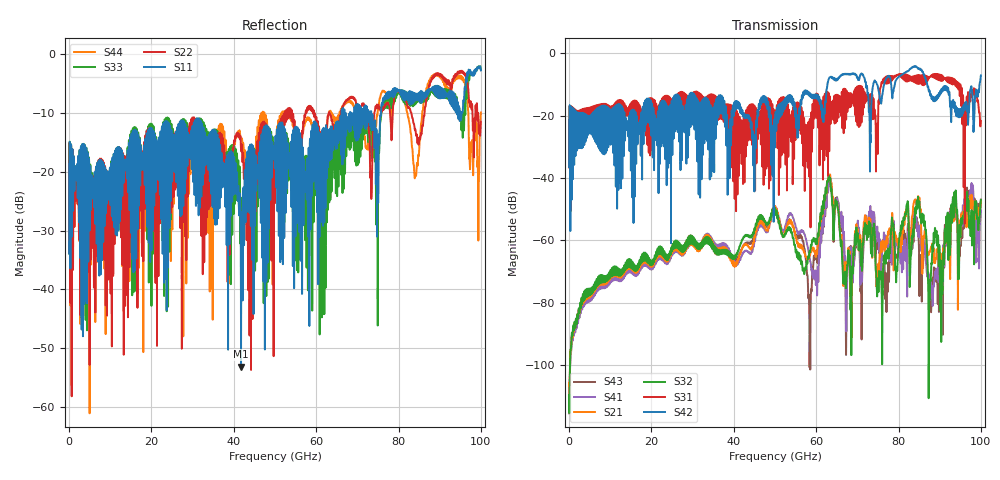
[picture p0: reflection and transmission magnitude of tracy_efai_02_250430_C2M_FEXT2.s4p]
!! PART DESCRIPTION: TE 224G+ VSR Channel- Chip to module, IO connector to CPC(Co-packaged connector) through over the board cable
!! CHANNEL DESCRIPTION: Module trace -> Mated IO 224G+ Connector -> Internal Cable Termination -> 30AWG 300mm Cable -> Cable
!!  termination + CPC connector(No footprint or package included)
!! MODEL REVISION:  Rev 3, Created on April 25, 2025
!! MODEL STATUS: Development
!! MODEL GEOMETRY: 8 Pair Channel
!! MODEL FREQUENCY RANGE: 0 GHz to 100 GHz in 10.00 MHz frequency steps
!! MODEL EDGE RATE LIMITATION: 5ps (Using conservative 0.5/Fmax rule of thumb)
!! PORT DEFINITIONS:
!! Port  1  ----->  Module Side  -->  Host Side, A Row  <-----  Port  2
!! Port  3  ----->  Module Side  -->  Host Side, A Row  <-----  Port  4
# GHz S MA R 45
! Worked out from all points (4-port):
!   10000 points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, 10 MHz to 100 GHz, reference 45 ohm
!   strongest paths, dB at 10 MHz, 25.01 GHz, 50.01 GHz, 75.01 GHz, 100 GHz:
!     S42: -36.5, -18.1, -28.3, -11.1, -7.2
!     S31: -36.7, -17.7, -20.3, -22.6, -21.7
!     S32: -115.0, -63.6, -49.7, -72.5, -47.1
!     S21: -112.4, -64.2, -49.2, -71.6, -47.8
!     S41: -115.1, -64.9, -49.3, -60.3, -50.4
!     S43: -115.4, -64.4, -49.9, -62.8, -46.9
!   lowest |S11| = -53.2 dB at 41.76 GHz (marker M1), VSWR 1.00, Z = 44.9 + j0.179 ohm
!   |S11| at or under -10 dB: start of sweep to 66.19 GHz; 67.15 GHz to 68.21 GHz (1.059 GHz wide, 1.57 % of centre); 73.39 GHz to 75.75 GHz (2.363 GHz wide, 3.17 % of centre)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
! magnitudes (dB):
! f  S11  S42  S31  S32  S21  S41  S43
! 10 MHz  -33.9  -36.5  -36.7  -115.0  -112.4  -115.1  -115.4
! 41.76 GHz  -53.2  -17.4  -22.0  -60.8  -63.5  -65.2  -63.1
! 58.47 GHz  -14.8  -12.8  -21.1  -63.6  -64.9  -66.4  -90.7
! 63.31 GHz  -13.0  -7.7  -14.0  -40.4  -39.4  -40.3  -41.2
! 66.95 GHz  -13.7  -6.8  -18.5  -72.6  -70.5  -66.7  -68.6
! 87.8 GHz  -5.9  -13.2  -7.5  -73.0  -62.7  -72.9  -80.2
! 100 GHz  -2.7  -7.2  -21.7  -47.1  -47.8  -50.4  -46.9
